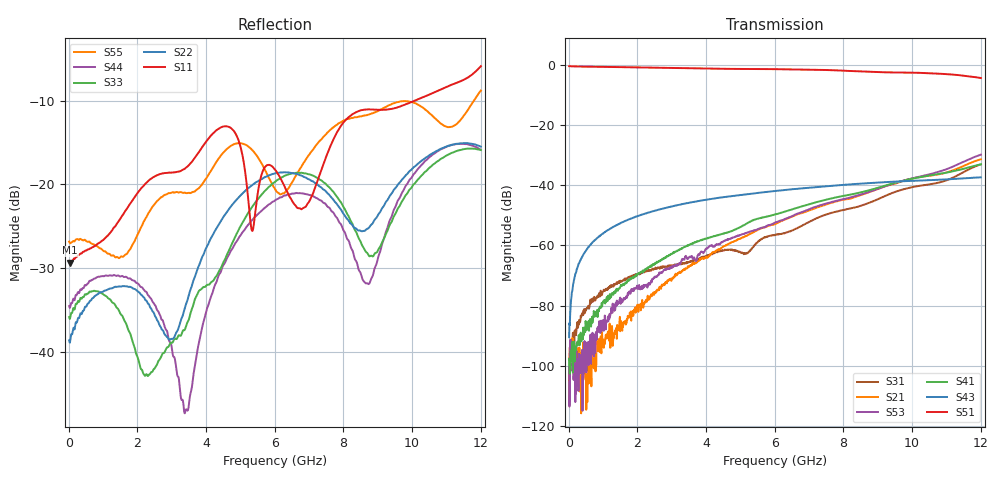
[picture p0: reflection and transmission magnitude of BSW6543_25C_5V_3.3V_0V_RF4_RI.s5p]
! Agilent Technologies	N5230C	MY49001333	A.09.33.09
!	Test time	=	2026-05-28 10:00
!	Product	=	BSW6543
!	Temp	=	25C
!	Logic	=	RF4
!	Port1	=	RFC
!	Port2	=	RF1
!	Port3	=	RF2
!	Port4	=	RF3
!	Port5	=	RF4
!S5P File: Measurements: <S11,S12,S13,S14,S15>,
!<S21,S22,S23,S24,S25>,
!<S31,S32,S33,S34,S35>,
!<S41,S42,S43,S44,S45>,
!<S51,S52,S53,S54,S55>;
# HZ S RI R 50
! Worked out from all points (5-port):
!   1201 points, 10 MHz to 12.01 GHz, reference 50 ohm
!   strongest paths, dB at 10 MHz, 3.01 GHz, 6.01 GHz, 9.01 GHz, 12.01 GHz:
!     S51: -0.5, -1.1, -1.4, -2.4, -4.4
!     S43: -90.5, -47.0, -41.9, -39.1, -37.4
!     S41: -97.7, -62.8, -49.7, -40.9, -33.1
!     S53: -98.3, -67.4, -52.5, -41.2, -29.8
!     S21: -101.0, -70.9, -52.9, -41.2, -31.4
!     S31: -112.9, -66.9, -56.6, -44.7, -33.1
!   lowest |S11| = -29.3 dB at 40 MHz (marker M1), VSWR 1.07, Z = 53.5 - j0.337 ohm
!   |S11| at or under -10 dB: start of sweep to 10.08 GHz
